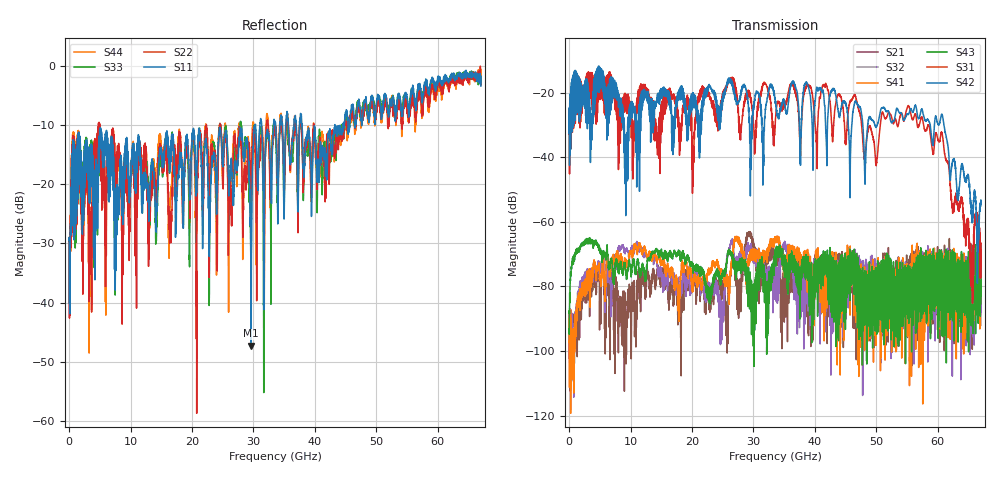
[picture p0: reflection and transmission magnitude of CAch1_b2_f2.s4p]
!Agilent Technologies,N5247A,US51170199,A.09.90.13
!Agilent N5247A: A.09.90.13
!Date: Thursday, October 18, 2018 09:55:04
!Correction: S11(Full 4 Port(1,2,3,4))
!S12(Full 4 Port(1,2,3,4))
!S13(Full 4 Port(1,2,3,4))
!S14(Full 4 Port(1,2,3,4))
!S21(Full 4 Port(1,2,3,4))
!S22(Full 4 Port(1,2,3,4))
!S23(Full 4 Port(1,2,3,4))
!S24(Full 4 Port(1,2,3,4))
!S31(Full 4 Port(1,2,3,4))
!S32(Full 4 Port(1,2,3,4))
!S33(Full 4 Port(1,2,3,4))
!S34(Full 4 Port(1,2,3,4))
!S41(Full 4 Port(1,2,3,4))
!S42(Full 4 Port(1,2,3,4))
!S43(Full 4 Port(1,2,3,4))
!S44(Full 4 Port(1,2,3,4))
!S4P File: Measurements: <S11,S12,S13,S14>,
!<S21,S22,S23,S24>,
!<S31,S32,S33,S34>,
!<S41,S42,S43,S44>:
# Hz S  dB  R 50
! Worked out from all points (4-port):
!   6701 points, 10 MHz to 67 GHz, reference 50 ohm
!   strongest paths, dB at 10 MHz, 16.76 GHz, 33.51 GHz, 50.25 GHz, 67 GHz:
!     S42: -32.6, -29.3, -21.5, -29.4, -54.2
!     S31: -32.9, -22.0, -30.8, -37.7, -66.8
!     S43: -93.2, -70.4, -72.5, -90.5, -77.6
!     S41: -90.1, -74.7, -66.5, -80.5, -71.0
!     S32: -97.2, -78.1, -80.8, -84.7, -77.4
!     S21: -88.1, -78.4, -71.7, -86.4, -70.3
!   lowest |S11| = -47.3 dB at 29.63 GHz (marker M1), VSWR 1.01, Z = 50.1 - j0.425 ohm
!   |S11| at or under -10 dB: start of sweep to 30.3 GHz; 31.33 GHz to 33.31 GHz (1.979 GHz wide, 6.12 % of centre); 37.9 GHz to 43.24 GHz (5.343 GHz wide, 13.2 % of centre)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
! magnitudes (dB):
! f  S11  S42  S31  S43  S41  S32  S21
! 10 MHz  -29.4  -32.6  -32.9  -93.2  -90.1  -97.2  -88.1
! 4.879 GHz  -12.2  -11.8  -16.7  -67.7  -72.7  -72.4  -76.9
! 9.269 GHz  -13.4  -40.9  -23.7  -75.5  -73.2  -68.4  -101.1
! 26.1 GHz  -20.1  -15.6  -16.7  -69.6  -80.3  -68.4  -77.7
! 29.63 GHz  -47.3  -40.1  -23.2  -79.5  -70.0  -68.2  -64.2
! 55.23 GHz  -8.1  -26.7  -24.1  -79.8  -78.3  -84.2  -75.8
! 67 GHz  -3.4  -54.2  -66.8  -77.6  -71.0  -77.4  -70.3
